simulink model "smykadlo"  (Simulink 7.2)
settings: Solver=ode45  StartTime=0.0  StopTime=0.2  RelTol=1e-3
InitFcn:
  | smykadlo_init;
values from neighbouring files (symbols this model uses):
  delka = 1    [smykadlo_init.m]
  delka2 = 0.5    [smykadlo_init.m]
  f1 = 0.1    [smykadlo_init.m]
  f2 = 0.1    [smykadlo_init.m]
  m = 1    [smykadlo_init.m]
  omega = 10    [smykadlo_init.m]
  uhel = fi*(pi/180)    (= 1.57079632679)    [smykadlo_init.m]
undefined symbols (not defined in the file or in its folder): deg, kg, N, rad, s
libraries: mblibv1 x13

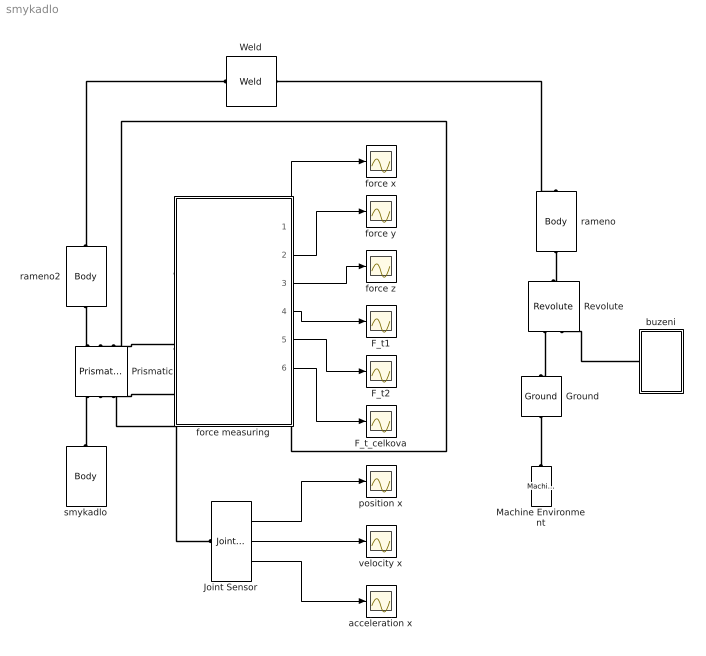
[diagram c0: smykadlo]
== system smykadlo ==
  " F_t1 " : Scope
  F_t2 : Scope
  F_t_celkova : Scope
  Ground : mblibv1/Bodies/Ground  Orientation=up  DialogController=MECH.DynMechDlgSource  SystemSampleTime=-1  UpdateFromCAD=off  LeftPortType=env  RightPortType=workingframe  PhysicalDomain=Mechanical  DialogClass=GroundBlock  CoordPosition=[0 0 0]  CoordPositionUnits=m  StateVectorMgrId=0  MachineId=[1 0]  ShowEnvPort=on
  Joint Sensor : mblibv1/Sensors &  Actuators/Joint Sensor  DialogController=MECH.DynMechDlgSource  SystemSampleTime=-1  UpdateFromCAD=off  PhysicalDomain=Mechanical  PortType=blob  Muxed=off  Pose=off  Angle=on  AngleUnits=deg  ArcVelocity=off  ArcVelocityUnits=deg/s  ArcAcceleration=off  ArcAccelerationUnits=deg/s^2  CoordPosition=on  CoordPositionUnits=m  Velocity=on  VelocityUnits=m/s  Acceleration=on  AccelerationUnits=m/s^2  Quaternion=on  QuaternionDT=off  QuaternionDDT=off  QuaternionUnits=off  OutputVector=[1]  ActiveIO=on  Width=3  DialogClass=MechanicalSensorBlock  Primitive=P1  Force=off  ForceUnits=N  Torque=off  TorqueUnits=N*m  ReferenceFrame=Absolute (World)  ReactionSensedSide=Base  ReactionReferenceFrame=Local (Body CS)  ReactionForce=off  ReactionForceUnits=N  ReactionMoment=off  ReactionMomentUnits=N*m
  Machine Environment : mblibv1/Bodies/Machine Environment  Orientation=up  DialogController=MECH.DialogSource  SystemSampleTime=-1  PortType=env  PhysicalDomain=Mechanical  DialogTemplateClass=MECH.MachineEnvironment  SyncWhenCopied=off  Gravity=[0 -9.81 0]  GravityUnits=m/s^2  GravityAsSignal=off  Dimensionality=Auto-detect  AnalysisType=Forward dynamics  LinearAssemblyTolerance=1e-3  LinearAssemblyToleranceUnits=m  AngularAssemblyTolerance=1e-3  AngularAssemblyToleranceUnits=rad  ConstraintSolverType=Stabilizing  ConstraintRelTolerance=1e-4  ConstraintAbsTolerance=1e-4  UseRobustSingularityHandling=off  RedundancyAnalysisToleranceType=Automatically select tolerance  RedundancyAnalysisTolerance=1e-14  StatePerturbationType=Fixed  PerturbationSize=1e-5  VisualizeMachine=on  BodyVisualizationType=Use model default body geometries  BodyColorSelMode=Use model default  DefaultBodyColor=[1 0 0]
  Prismatic : mblibv1/Joints/Prismatic  Orientation=down  DialogController=MECH.DynMechDlgSource  PhysicalDomain=mechanical  SubClassName=Unknown  LeftPortType=blob  RightPortType=blob  LConnTagsString=__newl0|SA1|SA2  RConnTagsString=__newr0|SA1|SA2  UpdateFromCAD=off  NumSAPorts=4  CutJoint=off  MarkAsCut=off  Primitives=prismatic  PrimitiveProps=P1$Base$[1 0 0]$prismatic  DialogClass=JointBlock  P1Axis=[1 0 0]
  Revolute : mblibv1/Joints/Revolute  Orientation=up  DialogController=MECH.DynMechDlgSource  PhysicalDomain=mechanical  SubClassName=Unknown  LeftPortType=blob  RightPortType=blob  LConnTagsString=__newl0|SA1  RConnTagsString=__newr0  UpdateFromCAD=off  NumSAPorts=1  CutJoint=off  MarkAsCut=off  Primitives=prismatic  PrimitiveProps=R1$World$[0 1 0]$revolute  DialogClass=JointBlock  R1Axis=[0 1 0]
  Weld : mblibv1/Joints/Weld  Orientation=left  DialogController=MECH.DynMechDlgSource  PhysicalDomain=mechanical  SubClassName=Unknown  LeftPortType=blob  RightPortType=blob  LConnTagsString=__newl0  RConnTagsString=__newr0  UpdateFromCAD=off  NumSAPorts=0  CutJoint=off  MarkAsCut=off  Primitives=weld  PrimitiveProps=W$WORLD$[0 0 0]$weld  DialogClass=JointBlock  WAxis=[0 0 0]
  acceleration x : Scope
  buzeni : Subsystem  Orientation=left
  force measuring : Subsystem
  force x : Scope
  force y : Scope
  force z : Scope
  position x : Scope
  rameno : mblibv1/Bodies/Body  Orientation=up  DialogController=MECH.DynMechDlgSource  PhysicalDomain=mechanical  SubClassName=Unknown  LeftPortType=workingframe  RightPortType=workingframe  LConnTagsString=CS1  RConnTagsString=CG  UpdateFromCAD=off  DialogClass=MechanicalBodyBlock  Mass=1  MassUnits=kg  InertiaUnits=kg*m^2  Inertia=eye(3)  Shape=Cylinder  ShapeDims=[1 1]  ShapeUnits=m  ShapeUse=false  Density=1  DensityUnits=kg/m^3  DensityUse=false  GraphicsMode=MACHINE_DEFAULT  BodyColorSelMode=MACHINE_DEFAULT  BodyColor=[1 0 0]  AttachedToCS=CG  CG=Right$CG$[0 delka 0]/2$CS1$CS1$m$[0 0 0]$Euler X-Y-Z$deg$WORLD$true$none  WorkingFrames=Left$CS1$[0 0 0]$Adjoining$Adjoining$m$[0 0 0]$Euler X-Y-Z$deg$WORLD$true$none#Right$CS2$[0 delka 0]$CS1$CS1$m$[0 0 0]$Euler X-Y-Z$deg$WORLD$false$none  CGPos=[0 delka 0]/2  CGRot=[0 0 0]  CS0Pos=[]  CS0Rot=[]  CS1Pos=[0 0 0]  CS1Rot=[0 0 0]  CS2Pos=[0 delka 0]  CS2Rot=[0 0 0]  CS3Pos=[]  CS3Rot=[]  CS4Pos=[]  CS4Rot=[]  CS5Pos=[]  CS5Rot=[]  CS6Pos=[]  CS6Rot=[]  CS7Pos=[]  CS7Rot=[]  CS8Pos=[]  CS8Rot=[]  CS9Pos=[]  CS9Rot=[]  CS10Pos=[]  CS10Rot=[]  CS11Pos=[]  CS11Rot=[]  CS12Pos=[]  CS12Rot=[]  CS13Pos=[]  CS13Rot=[]  CS14Pos=[]  CS14Rot=[]  CS15Pos=[]  CS15Rot=[]  CS16Pos=[]  CS16Rot=[]  CS17Pos=[]  CS17Rot=[]  CS18Pos=[]  CS18Rot=[]  CS19Pos=[]  CS19Rot=[]  CS20Pos=[]  CS20Rot=[]
  rameno2 : mblibv1/Bodies/Body  Orientation=down  DialogController=MECH.DynMechDlgSource  PhysicalDomain=mechanical  SubClassName=Unknown  LeftPortType=workingframe  RightPortType=workingframe  LConnTagsString=CS1  RConnTagsString=CG  UpdateFromCAD=off  DialogClass=MechanicalBodyBlock  Mass=1  MassUnits=kg  InertiaUnits=kg*m^2  Inertia=eye(3)  Shape=Cylinder  ShapeDims=[1 1]  ShapeUnits=m  ShapeUse=false  Density=1  DensityUnits=kg/m^3  DensityUse=false  GraphicsMode=MACHINE_DEFAULT  BodyColorSelMode=MACHINE_DEFAULT  BodyColor=[1 0 0]  AttachedToCS=CG  CG=Right$CG$[-sin(uhel)*delka2 -cos(uhel)*delka2 0]/2$World$CS1$m$[0 0 90-fi]$Euler X-Y-Z$deg$World$true$none  WorkingFrames=Left$CS1$[0 0 0]$World$Adjoining$m$[0 0 90-fi]$Euler X-Y-Z$deg$World$true$none#Right$CS2$[-sin(uhel)*delka2 -cos(uhel)*delka2 0]$World$CS1$m$[0 0 90-fi]$Euler X-Y-Z$deg$World$false$none  CGPos=[-sin(uhel)*delka2 -cos(uhel)*delka2 0]/2  CGRot=[0 0 90-fi]  CS0Pos=[]  CS0Rot=[]  CS1Pos=[0 0 0]  CS1Rot=[0 0 90-fi]  CS2Pos=[-sin(uhel)*delka2 -cos(uhel)*delka2 0]  CS2Rot=[0 0 90-fi]  CS3Pos=[]  CS3Rot=[]  CS4Pos=[]  CS4Rot=[]  CS5Pos=[]  CS5Rot=[]  CS6Pos=[]  CS6Rot=[]  CS7Pos=[]  CS7Rot=[]  CS8Pos=[]  CS8Rot=[]  CS9Pos=[]  CS9Rot=[]  CS10Pos=[]  CS10Rot=[]  CS11Pos=[]  CS11Rot=[]  CS12Pos=[]  CS12Rot=[]  CS13Pos=[]  CS13Rot=[]  CS14Pos=[]  CS14Rot=[]  CS15Pos=[]  CS15Rot=[]  CS16Pos=[]  CS16Rot=[]  CS17Pos=[]  CS17Rot=[]  CS18Pos=[]  CS18Rot=[]  CS19Pos=[]  CS19Rot=[]  CS20Pos=[]  CS20Rot=[]
  smykadlo : mblibv1/Bodies/Body  Orientation=down  DialogController=MECH.DynMechDlgSource  PhysicalDomain=mechanical  SubClassName=Unknown  LeftPortType=workingframe  RightPortType=workingframe  LConnTagsString=CG  UpdateFromCAD=off  DialogClass=MechanicalBodyBlock  Mass=m  MassUnits=kg  InertiaUnits=kg*m^2  Inertia=eye(3)  Shape=Cylinder  ShapeDims=[1 1]  ShapeUnits=m  ShapeUse=false  Density=1  DensityUnits=kg/m^3  DensityUse=false  GraphicsMode=MACHINE_DEFAULT  BodyColorSelMode=MACHINE_DEFAULT  BodyColor=[1 0 0]  AttachedToCS=CG  CG=Left$CG$[0 0 0]$Adjoining$Adjoining$m$[0 0 0]$Euler X-Y-Z$deg$Adjoining$true$none  WorkingFrames=Right$CS1$[0 0 0]$CG$CG$m$[0 0 0]$Euler X-Y-Z$deg$CG$false$none  CGPos=[0 0 0]  CGRot=[0 0 0]  CS0Pos=[]  CS0Rot=[]  CS1Pos=[0 0 0]  CS1Rot=[0 0 0]  CS2Pos=[]  CS2Rot=[]  CS3Pos=[]  CS3Rot=[]  CS4Pos=[]  CS4Rot=[]  CS5Pos=[]  CS5Rot=[]  CS6Pos=[]  CS6Rot=[]  CS7Pos=[]  CS7Rot=[]  CS8Pos=[]  CS8Rot=[]  CS9Pos=[]  CS9Rot=[]  CS10Pos=[]  CS10Rot=[]  CS11Pos=[]  CS11Rot=[]  CS12Pos=[]  CS12Rot=[]  CS13Pos=[]  CS13Rot=[]  CS14Pos=[]  CS14Rot=[]  CS15Pos=[]  CS15Rot=[]  CS16Pos=[]  CS16Rot=[]  CS17Pos=[]  CS17Rot=[]  CS18Pos=[]  CS18Rot=[]  CS19Pos=[]  CS19Rot=[]  CS20Pos=[]  CS20Rot=[]
  velocity x : Scope
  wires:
  force measuring/1(Fr_x) -> force x/1
  force measuring/4(F_t1) -> " F_t1 "/1
  force measuring/5(F_t2) -> F_t2/1
  force measuring/2(F_n1) -> force y/1
  force measuring/3(F_n2) -> force z/1
  Joint Sensor/1 -> position x/1
  Joint Sensor/3 -> acceleration x/1
  Joint Sensor/2 -> velocity x/1
  force measuring/6(F_t_celk) -> F_t_celkova/1
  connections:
  Revolute/LConn1 -- Ground/RConn1
  rameno/LConn1 -- Revolute/RConn1
  Weld/LConn1 -- rameno/RConn1
  rameno2/LConn1 -- Weld/RConn1
  smykadlo/LConn1 -- Prismatic/RConn1
  buzeni/RConn1 -- Revolute/LConn2
  rameno2/RConn1 -- Prismatic/LConn1
  force measuring/LConn1 -- Prismatic/LConn3
  Machine Environment/RConn1 -- Ground/LConn1
  force measuring/LConn2 -- Prismatic/RConn3
  Joint Sensor/LConn1 -- Prismatic/RConn2
  force measuring/RConn1 -- Prismatic/LConn2

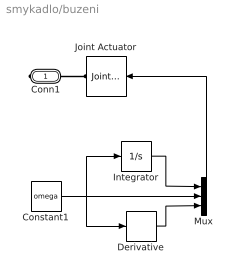
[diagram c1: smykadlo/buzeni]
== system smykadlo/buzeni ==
  Constant1 : Constant  Value=omega  OutDataType=sfix(16)  OutScaling=2^0
  Derivative : Derivative
  Integrator : Integrator
  Joint Actuator : mblibv1/Sensors &  Actuators/Joint Actuator  Orientation=left  DialogController=MECH.DynMechDlgSource  SystemSampleTime=-1  UpdateFromCAD=off  PhysicalDomain=Mechanical  PortType=blob  ActuationStyle=Motion  AngleUnits=rad  ArcVelocityUnits=rad/s  ArcAccelerationUnits=rad/s^2  CoordPositionUnits=m  VelocityUnits=m/s  AccelerationUnits=m/s^2  ForceUnits=N  TorqueUnits=N*m  ActiveIO=on  Width=3  DialogClass=MechanicalActuatorBlock  Primitive=R1  ReferenceFrame=Absolute (World)
  Mux : Mux  Inputs=3
  Conn1 : PMIOPort  Port=1  Side=Right
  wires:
  Mux/1 -> Joint Actuator/1
  Derivative/1 -> Mux/3
  Integrator/1 -> Mux/1
  Constant1/1 -> Derivative/1, Mux/2, Integrator/1
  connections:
  Conn1/RConn1 -- Joint Actuator/RConn1

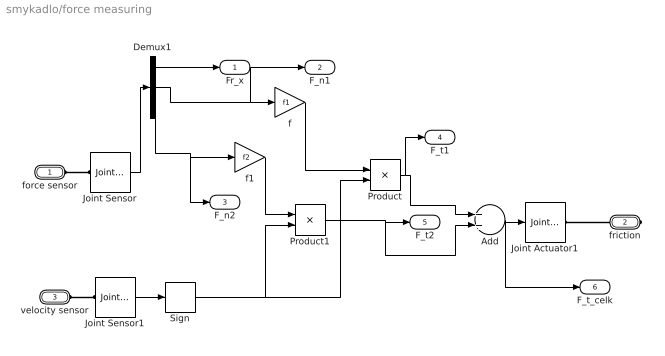
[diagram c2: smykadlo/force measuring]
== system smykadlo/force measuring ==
  Add : Sum  OutDataType=sfix(16)  OutScaling=2^-10
  Demux1 : Demux  Outputs=3
  Joint Actuator1 : mblibv1/Sensors &  Actuators/Joint Actuator  DialogController=MECH.DynMechDlgSource  SystemSampleTime=-1  UpdateFromCAD=off  PhysicalDomain=Mechanical  PortType=blob  ActuationStyle=Force  AngleUnits=deg  ArcVelocityUnits=deg/s  ArcAccelerationUnits=deg/s^2  CoordPositionUnits=m  VelocityUnits=m/s  AccelerationUnits=m/s^2  ForceUnits=N  TorqueUnits=N-m  ActiveIO=on  Width=1  DialogClass=MechanicalActuatorBlock  Primitive=P1  ReferenceFrame=Absolute (World)
  Joint Sensor : mblibv1/Sensors &  Actuators/Joint Sensor  DialogController=MECH.DynMechDlgSource  SystemSampleTime=-1  UpdateFromCAD=off  PhysicalDomain=Mechanical  PortType=blob  Muxed=off  Pose=off  Angle=on  AngleUnits=deg  ArcVelocity=off  ArcVelocityUnits=deg/s  ArcAcceleration=off  ArcAccelerationUnits=deg/s^2  CoordPosition=off  CoordPositionUnits=m  Velocity=off  VelocityUnits=m/s  Acceleration=off  AccelerationUnits=m/s^2  Quaternion=on  QuaternionDT=off  QuaternionDDT=off  QuaternionUnits=off  OutputVector=[1]  ActiveIO=on  Width=3  DialogClass=MechanicalSensorBlock  Primitive=P1  Force=off  ForceUnits=N  Torque=off  TorqueUnits=N*m  ReferenceFrame=Absolute (World)  ReactionSensedSide=Base  ReactionReferenceFrame=Local (Body CS)  ReactionForce=on  ReactionForceUnits=N  ReactionMoment=off  ReactionMomentUnits=N*m
  Joint Sensor1 : mblibv1/Sensors &  Actuators/Joint Sensor  DialogController=MECH.DynMechDlgSource  SystemSampleTime=-1  UpdateFromCAD=off  PhysicalDomain=Mechanical  PortType=blob  Muxed=off  Pose=off  Angle=on  AngleUnits=deg  ArcVelocity=off  ArcVelocityUnits=deg/s  ArcAcceleration=off  ArcAccelerationUnits=deg/s^2  CoordPosition=off  CoordPositionUnits=m  Velocity=on  VelocityUnits=m/s  Acceleration=off  AccelerationUnits=m/s^2  Quaternion=on  QuaternionDT=off  QuaternionDDT=off  QuaternionUnits=off  OutputVector=[1]  ActiveIO=on  Width=1  DialogClass=MechanicalSensorBlock  Primitive=P1  Force=off  ForceUnits=N  Torque=off  TorqueUnits=N*m  ReferenceFrame=Absolute (World)  ReactionSensedSide=Base  ReactionReferenceFrame=Local (Body CS)  ReactionForce=off  ReactionForceUnits=N  ReactionMoment=off  ReactionMomentUnits=N*m
  Product : Product  OutDataType=sfix(16)  OutScaling=2^0
  Product1 : Product  OutDataType=sfix(16)  OutScaling=2^0
  Sign : Signum
  f : Gain  Gain=f1  ParameterDataType=sfix(16)  ParameterScaling=2^0  OutDataType=sfix(16)  OutScaling=2^0
  f1 : Gain  Gain=f2  ParameterDataType=sfix(16)  ParameterScaling=2^0  OutDataType=sfix(16)  OutScaling=2^0
  force sensor : PMIOPort  Port=1  Side=Left
  friction : PMIOPort  Orientation=left  Port=2  Side=Right
  velocity sensor : PMIOPort  Port=3  Side=Left
  Fr_x : Outport
  F_n1 : Outport  Port=2
  F_n2 : Outport  Port=3
  F_t1 : Outport  Port=4
  F_t2 : Outport  Port=5
  F_t_celk : Outport  Port=6
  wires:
  Joint Sensor1/1 -> Sign/1
  Demux1/2 -> f/1, F_n1/1
  Demux1/3 -> f1/1, F_n2/1
  Joint Sensor/1 -> Demux1/1
  f/1 -> Product/1
  f1/1 -> Product1/1
  Sign/1 -> Product1/2, Product/2
  Product1/1 -> Add/2, F_t2/1
  Product/1 -> Add/1, F_t1/1
  Add/1 -> Joint Actuator1/1, F_t_celk/1
  Demux1/1 -> Fr_x/1
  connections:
  force sensor/RConn1 -- Joint Sensor/LConn1
  friction/RConn1 -- Joint Actuator1/RConn1
  velocity sensor/RConn1 -- Joint Sensor1/LConn1
